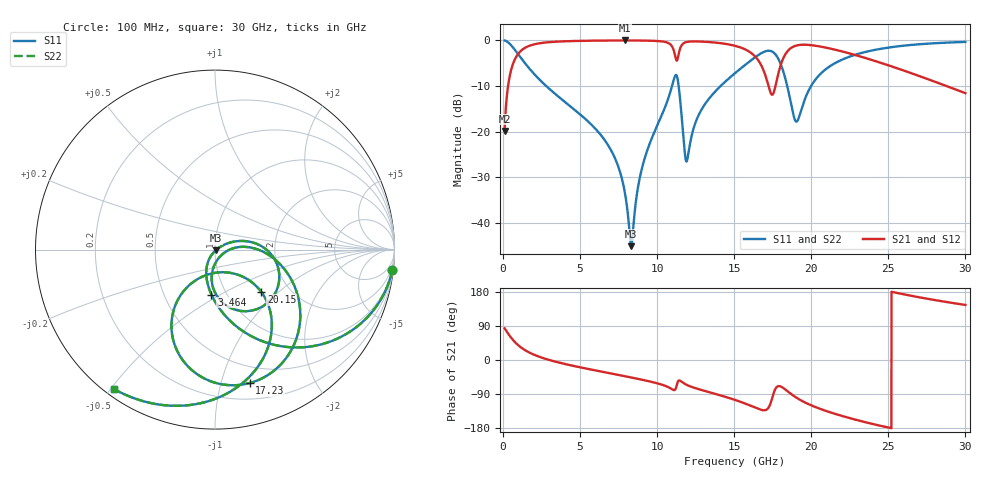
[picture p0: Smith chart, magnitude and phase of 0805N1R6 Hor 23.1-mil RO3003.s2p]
# GHz S MA R 50
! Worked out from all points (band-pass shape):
!   3201 points, 100 MHz to 30 GHz, reference 50 ohm
!   highest |S21| = -0.05 dB at 7.902 GHz (marker M1); lowest = -19.8 dB at 100 MHz (marker M2)
!   |S21| within 3 dB of the highest: 964.6 MHz to 11.14 GHz (10.18 GHz wide, 168 % of centre); 11.39 GHz to 16.2 GHz (4.804 GHz wide, 34.8 % of centre)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
!   lowest |S11| = -45.1 dB at 8.313 GHz (marker M3), VSWR 1.01, Z = 50.4 - j0.427 ohm
!   |S11| at or under -10 dB: 2.794 GHz to 10.96 GHz (8.171 GHz wide, 119 % of centre); 11.39 GHz to 14.12 GHz (2.729 GHz wide, 21.4 % of centre); 18.44 GHz to 19.99 GHz (1.552 GHz wide, 8.08 % of centre)
!   |S22| runs from -45.1 to 0.0 dB; largest |S21 - S12| = 0
!   S11 on the Smith chart (normalised r, x): 100 MHz: 1, -18; 3.464 GHz: 0.85, -0.46; 17.23 GHz: 0.34, -1.24; 20.15 GHz: 1.45, -0.78; 30 GHz: 0.03, -0.51
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0.1  0.9948 -6.4  0.1019 83.6  0.1019 83.6  0.9948 -6.4
0.436375  0.9126 -26.6  0.4084 63.4  0.4084 63.4  0.9126 -26.6
0.92225  0.725 -48.7  0.6878 41.2  0.6878 41.2  0.725 -48.7
3.46375  0.252 -94.5  0.965 -5.1  0.965 -5.1  0.252 -94.5
5.089563  0.1502 -108.8  0.9852 -20.1  0.9852 -20.1  0.1502 -108.8
6.967656  0.06432 -121.4  0.9933 -35.3  0.9933 -35.3  0.06432 -121.4
7.902031  0.0216 -119.0  0.9944 -42.7  0.9944 -42.7  0.0216 -119.0
8.313156  0.005584 -49.4  0.9941 -46.1  0.9941 -46.1  0.005584 -49.4
8.976562  0.0376 28.0  0.9923 -51.7  0.9923 -51.7  0.0376 28.0
10.06978  0.1237 21.8  0.9793 -62.3  0.9793 -62.3  0.1237 21.8
11.22841  0.4174 -43.9  0.6133 -72.6  0.6133 -72.6  0.4174 -43.9
11.93853  0.04847 -33.2  0.9585 -66.1  0.9585 -66.1  0.04847 -33.2
12.88225  0.1747 4.9  0.9664 -79.2  0.9664 -79.2  0.1747 4.9
15.05  0.4363 -19.3  0.8696 -105.3  0.8696 -105.3  0.4363 -19.3
16.41419  0.662 -46.0  0.6478 -126.6  0.6478 -126.6  0.662 -46.0
17.22709  0.7682 -75.4  0.3147 -125.6  0.3147 -125.6  0.7682 -75.4
18.04934  0.5299 -116.8  0.5569 -70.5  0.5569 -70.5  0.5299 -116.8
19.00241  0.129 -88.2  0.8722 -98.6  0.8722 -98.6  0.129 -88.2
20.03956  0.3266 -41.8  0.8819 -120.4  0.8819 -120.4  0.3266 -41.8
20.15169  0.3489 -42.4  0.877 -122.3  0.877 -122.3  0.3489 -42.4
25.01978  0.832 -90.0  0.5306 -178.4  0.5306 -178.4  0.832 -90.0
30  0.9588 -125.8  0.2635 145.3  0.2635 145.3  0.9588 -125.8
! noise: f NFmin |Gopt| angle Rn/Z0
0.1  0.001032  0.9443  1.577  0.004143
3.417  0.007169  0.7352  20.13  0.005248
6.743  0.01265  0.7138  37.99  0.007824
10.06  0.02635  0.7922  54.97  0.02066
13.39  0.03533  0.8  71.29  0.02433
16.7  0.1595  0.9423  86.95  0.3256
20.03  0.08443  0.877  101.5  0.0598
23.35  0.06903  0.8339  114.3  0.02633
26.67  0.07909  0.8402  126.6  0.02179
30  0.1011  0.8646  138.7  0.02067
